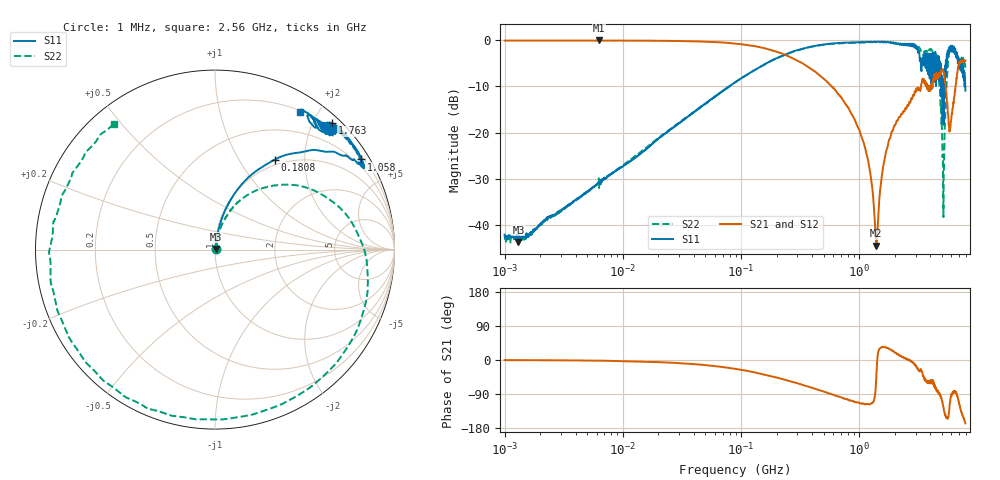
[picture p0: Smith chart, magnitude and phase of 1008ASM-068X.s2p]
!s-Parameter Generated by FASTRON Sdn. Bhd.
!FASTRON P/N : 1008ASM-068X
!Keysight Technologies: E5071C_MY46733604_B.14.02
!Date: Tue Nov 21 11:32:34 2023
!Version  :Rev00  Wed Nov 22 15:51:42 2023
!Data & Calibration Information:
!Freq  S11:SOLT2(ON)  S21:SOLT2(ON)  S12:SOLT2(ON)  S22:SOLT2(ON)
!PortZ  Port1:50+j0  Port2:50+j0
!When reading reference impedance value at option line is always used.
! Remarks : This data is being provided solely for informational purposes.
# Hz S dB R 50
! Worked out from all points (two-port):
!   1599 points, 1 MHz to 7.923 GHz, reference 50 ohm
!   highest |S21| = -0.03 dB at 6.301 MHz (marker M1); lowest = -44.5 dB at 1.396 GHz (marker M2)
!   |S21| within 3 dB of the highest: start of sweep to 230.3 MHz
!   lowest |S11| = -43.7 dB at 1.31 MHz (marker M3), VSWR 1.01, Z = 50.6 + j0.356 ohm
!   |S11| at or under -10 dB: start of sweep to 79.12 MHz; 4.154024 GHz to 4.158076 GHz (4.052 MHz wide, 0.0975 % of centre); 5.036 GHz to 5.218 GHz (182.2 MHz wide, 3.55 % of centre)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
!   |S22| runs from -44.6 to -0.3 dB; largest |S21 - S12| = 0.011
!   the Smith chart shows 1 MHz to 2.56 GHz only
!   S11 on the Smith chart (normalised r, x): 1 MHz: 1.01, +0.01; 180.8 MHz: 0.92, +1.44; 1.058 GHz: 0.29, +3.51; 1.763 GHz: 0.13, +2.28; 2.56 GHz: 0.22, +1.77
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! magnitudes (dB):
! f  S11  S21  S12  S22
! 1 MHz  -42.1  -0.1  -0.1  -42.2
! 1.31 MHz  -43.7  -0.1  -0.1  -44.6
! 4.479 MHz  -33.7  -0.1  -0.1  -33.7
! 6.301 MHz  -30.9  0.0  -0.1  -32.0
! 19.95 MHz  -21.3  -0.1  -0.1  -21.2
! 89.01 MHz  -9.1  -0.7  -0.7  -9.1
! 180.8 MHz  -4.4  -2.1  -2.1  -4.4
! 398.5 MHz  -1.3  -6.3  -6.3  -1.4
! 715.4 MHz  -0.6  -12.6  -12.6  -0.6
! 1.058 GHz  -0.4  -21.3  -21.3  -0.5
! 1.234 GHz  -0.3  -28.3  -28.3  -0.4
! 1.396 GHz  -0.4  -44.5  -44.6  -0.4
! 1.566 GHz  -0.3  -28.8  -28.8  -0.4
! 1.763 GHz  -0.4  -22.3  -22.3  -0.5
! 1.784 GHz  -0.5  -21.7  -21.7  -0.5
! 2.56 GHz  -0.9  -14.0  -14.1  -0.9
! 4.437 GHz  -5.1  -8.5  -8.5  -3.2
! 4.717 GHz  -3.5  -7.7  -7.7  -7.3
! 5.136 GHz  -11.2  -6.5  -6.5  -31.6
! 5.841 GHz  -2.2  -19.5  -19.5  -1.7
! 6.959 GHz  -4.8  -5.2  -5.2  -4.2
! 7.923 GHz  -10.9  -4.5  -4.4  -6.7
